(* Logix 5000 AddOnInstructionDefinition export NTEC_VerifyLimits; software revision ?; part 2 of 2 *)
(* tags used below, declared in another part *)
   NTEC_Axis : NTEC_Axis;   // NTEC Axis Tag
   EN : BOOL;   // Enabled
   DN : BOOL;   // Successfully Done
   ERR : BOOL;   // Instruction Error
   ERR_Code : DINT;   // Instruction Error Code
   State : DINT;
   Enable : BOOL;
(* NTEC_VerifyLimits, continued *)

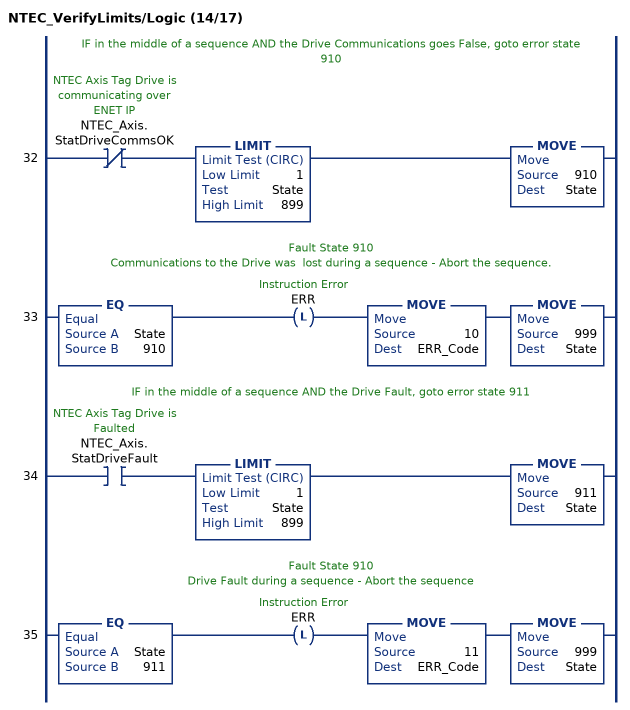
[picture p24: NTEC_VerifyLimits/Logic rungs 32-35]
   // IF in the middle of a sequence AND the Drive Communications goes False, goto error state 910
   32: XIO(NTEC_Axis.StatDriveCommsOK)LIMIT(1,State,899)MOVE(910,State);
   // Fault State 910
   // Communications to the Drive was  lost during a sequence - Abort the sequence.
   33: EQ(State,910)OTL(ERR)MOVE(10,ERR_Code)MOVE(999,State);
   // IF in the middle of a sequence AND the Drive Fault, goto error state 911
   34: XIC(NTEC_Axis.StatDriveFault)LIMIT(1,State,899)MOVE(911,State);
   // Fault State 910
   // Drive Fault during a sequence - Abort the sequence
   35: EQ(State,911)OTL(ERR)MOVE(11,ERR_Code)MOVE(999,State);
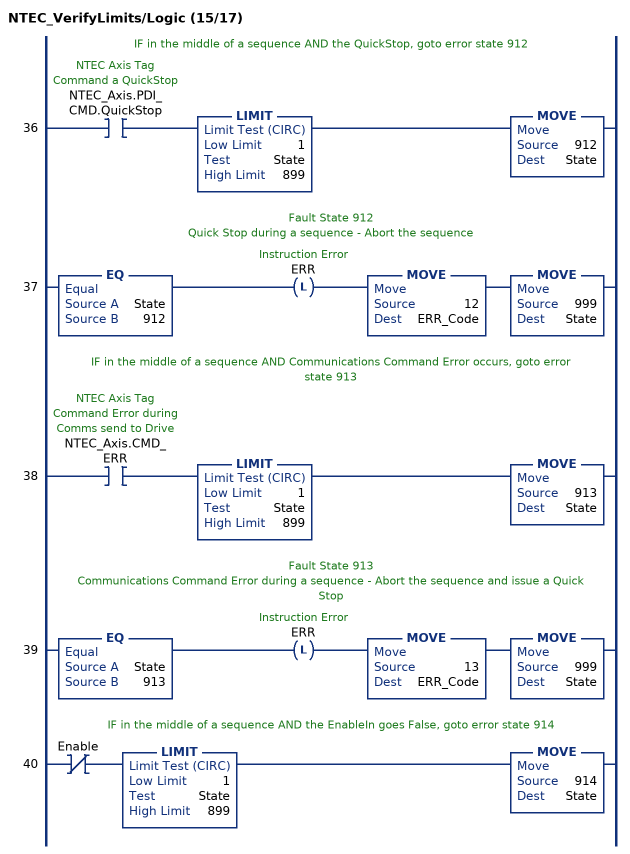
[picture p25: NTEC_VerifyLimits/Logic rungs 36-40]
   // IF in the middle of a sequence AND the QuickStop, goto error state 912
   36: XIC(NTEC_Axis.PDI_CMD.QuickStop)LIMIT(1,State,899)MOVE(912,State);
   // Fault State 912
   // Quick Stop during a sequence - Abort the sequence
   37: EQ(State,912)OTL(ERR)MOVE(12,ERR_Code)MOVE(999,State);
   // IF in the middle of a sequence AND Communications Command Error occurs, goto error state 913
   38: XIC(NTEC_Axis.CMD_ERR)LIMIT(1,State,899)MOVE(913,State);
   // Fault State 913
   // Communications Command Error during a sequence - Abort the sequence and issue a Quick Stop
   39: EQ(State,913)OTL(ERR)MOVE(13,ERR_Code)MOVE(999,State);
   // IF in the middle of a sequence AND the EnableIn goes False, goto error state 914
   40: XIO(Enable)LIMIT(1,State,899)MOVE(914,State);
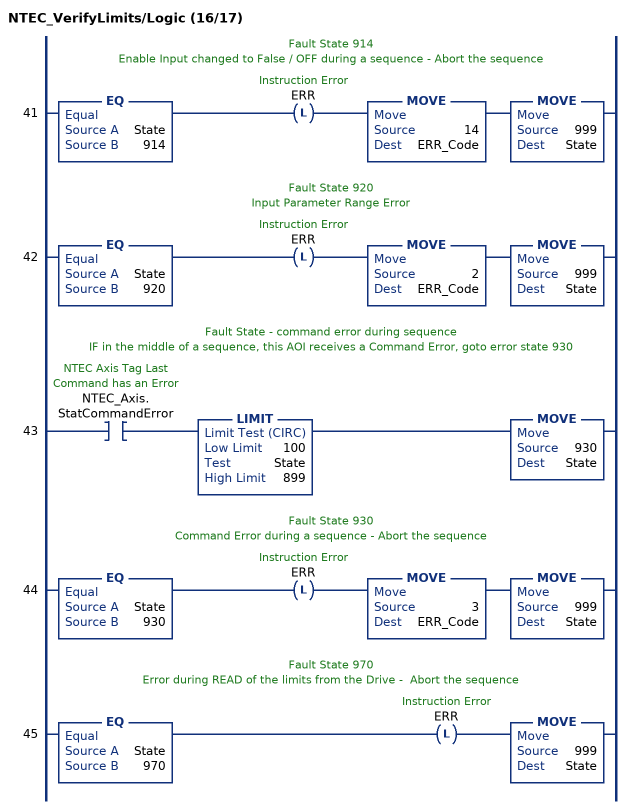
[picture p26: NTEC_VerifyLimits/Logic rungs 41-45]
   // Fault State 914
   // Enable Input changed to False / OFF during a sequence - Abort the sequence
   41: EQ(State,914)OTL(ERR)MOVE(14,ERR_Code)MOVE(999,State);
   // Fault State 920
   // Input Parameter Range Error
   42: EQ(State,920)OTL(ERR)MOVE(2,ERR_Code)MOVE(999,State);
   // Fault State - command error during sequence
   // IF in the middle of a sequence, this AOI receives a Command Error, goto error state 930
   43: XIC(NTEC_Axis.StatCommandError)LIMIT(100,State,899)MOVE(930,State);
   // Fault State 930
   // Command Error during a sequence - Abort the sequence
   44: EQ(State,930)OTL(ERR)MOVE(3,ERR_Code)MOVE(999,State);
   // Fault State 970
   // Error during READ of the limits from the Drive -  Abort the sequence
   45: EQ(State,970)OTL(ERR)MOVE(999,State);
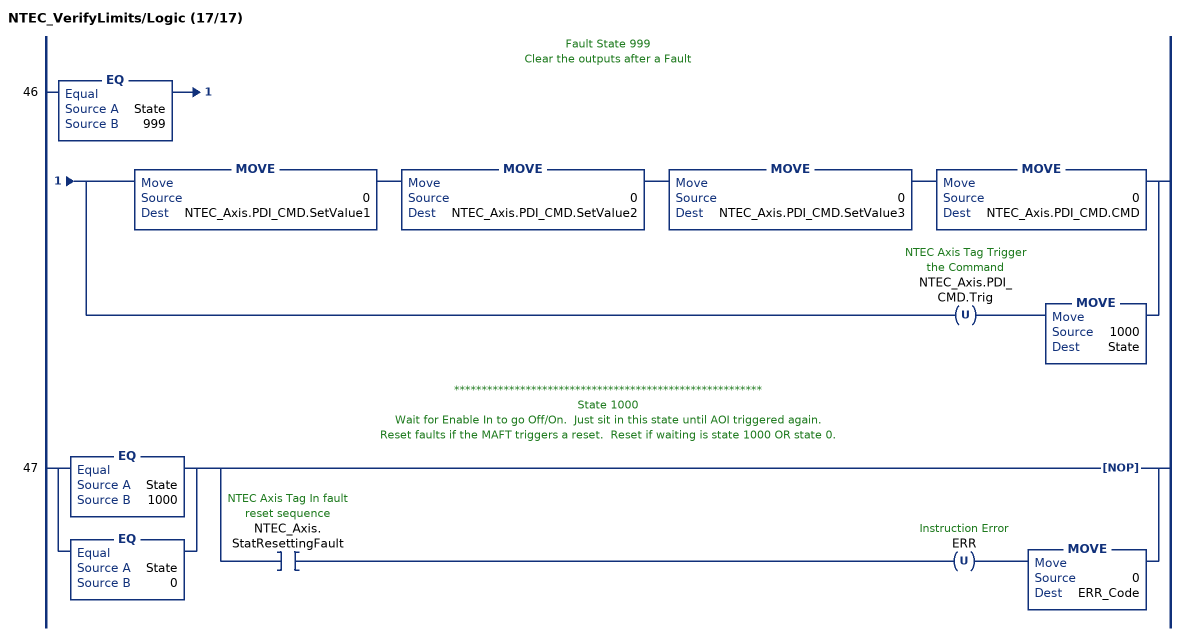
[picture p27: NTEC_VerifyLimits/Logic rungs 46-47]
   // Fault State 999
   // Clear the outputs after a Fault
   46: EQ(State,999)[MOVE(0,NTEC_Axis.PDI_CMD.SetValue1) MOVE(0,NTEC_Axis.PDI_CMD.SetValue2) MOVE(0,NTEC_Axis.PDI_CMD.SetValue3) MOVE(0,NTEC_Axis.PDI_CMD.CMD) ,OTU(NTEC_Axis.PDI_CMD.Trig) MOVE(1000,State) ];
   // ********************************************************
   // State 1000
   // Wait for Enable In to go Off/On.  Just sit in this state until AOI triggered again.
   // Reset faults if the MAFT triggers a reset.  Reset if waiting is state 1000 OR state 0.
   47: [EQ(State,1000) ,EQ(State,0) ][NOP() ,XIC(NTEC_Axis.StatResettingFault) OTU(ERR) MOVE(0,ERR_Code) ];
END_ROUTINE

ROUTINE Postscan   (* ladder *)
// Home Post-Scan Routine
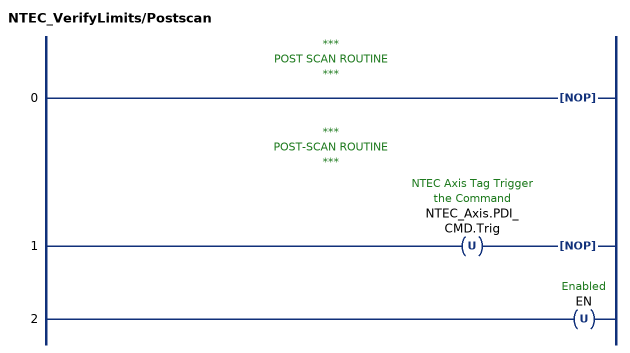
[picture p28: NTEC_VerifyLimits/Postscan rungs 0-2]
   // ***
   // POST SCAN ROUTINE
   // ***
   0: NOP();
   // ***
   // POST-SCAN ROUTINE
   // ***
   1: OTU(NTEC_Axis.PDI_CMD.Trig)NOP();
   2: OTU(EN);
END_ROUTINE

ROUTINE Prescan   (* ladder *)
// Home Pre-Scan Routine
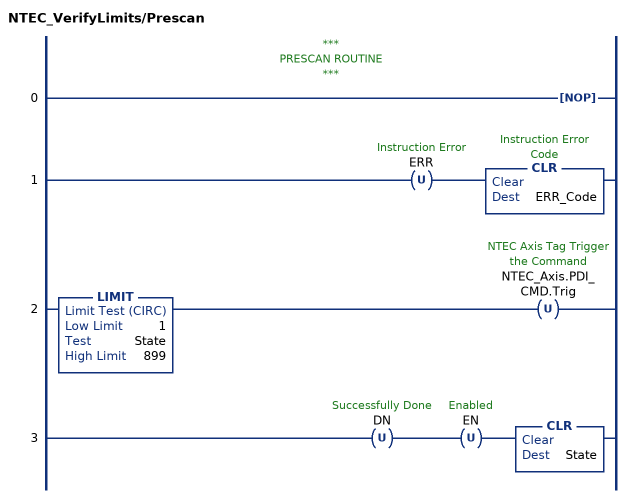
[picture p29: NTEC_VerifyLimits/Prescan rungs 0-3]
   // ***
   // PRESCAN ROUTINE
   // ***
   0: NOP();
   1: OTU(ERR)CLR(ERR_Code);
   2: LIMIT(1,State,899)OTU(NTEC_Axis.PDI_CMD.Trig);
   3: OTU(DN)OTU(EN)CLR(State);
END_ROUTINE
END_ADD_ON_INSTRUCTION
